FUNCTION_BLOCK FB_LD_IEDLD1 EXTENDS FB_AcsiCommonLogicalDeviceClass
VAR_INPUT
	LLN0: FB_LN_IED_LD1_LLN0 := (sClass:='LLN0', bLinkResult:=THIS^.AddLogicalNodeToContainer(ipLogicalNode:=LLN0));
	LPHD1: FB_LN_IED_LD1_LPHD1 := (sClass:='LPHD', bLinkResult:=THIS^.AddLogicalNodeToContainer(ipLogicalNode:=LPHD1));
	MMXU1: FB_LN_IED_LD1_MMXU1 := (sClass:='MMXU', bLinkResult:=THIS^.AddLogicalNodeToContainer(ipLogicalNode:=MMXU1));
	XCBR1: FB_LN_IED_LD1_XCBR1 := (sClass:='XCBR', bLinkResult:=THIS^.AddLogicalNodeToContainer(ipLogicalNode:=XCBR1));
	CSWI1: FB_LN_IED_LD1_CSWI1 := (sClass:='CSWI', bLinkResult:=THIS^.AddLogicalNodeToContainer(ipLogicalNode:=CSWI1));
	LEDGGIO1: FB_LN_IED_LD1_LEDGGIO1 := (sClass:='GGIO', bLinkResult:=THIS^.AddLogicalNodeToContainer(ipLogicalNode:=LEDGGIO1));
	LEDGGIO2: FB_LN_IED_LD1_LEDGGIO2 := (sClass:='GGIO', bLinkResult:=THIS^.AddLogicalNodeToContainer(ipLogicalNode:=LEDGGIO2));
	LEDGGIO3: FB_LN_IED_LD1_LEDGGIO3 := (sClass:='GGIO', bLinkResult:=THIS^.AddLogicalNodeToContainer(ipLogicalNode:=LEDGGIO3));
	LEDGGIO4: FB_LN_IED_LD1_LEDGGIO4 := (sClass:='GGIO', bLinkResult:=THIS^.AddLogicalNodeToContainer(ipLogicalNode:=LEDGGIO4));
	LEDGGIO5: FB_LN_IED_LD1_LEDGGIO5 := (sClass:='GGIO', bLinkResult:=THIS^.AddLogicalNodeToContainer(ipLogicalNode:=LEDGGIO5));
	LEDGGIO6: FB_LN_IED_LD1_LEDGGIO6 := (sClass:='GGIO', bLinkResult:=THIS^.AddLogicalNodeToContainer(ipLogicalNode:=LEDGGIO6));
	LEDGGIO7: FB_LN_IED_LD1_LEDGGIO7 := (sClass:='GGIO', bLinkResult:=THIS^.AddLogicalNodeToContainer(ipLogicalNode:=LEDGGIO7));
	LEDGGIO8: FB_LN_IED_LD1_LEDGGIO8 := (sClass:='GGIO', bLinkResult:=THIS^.AddLogicalNodeToContainer(ipLogicalNode:=LEDGGIO8));
	ATCC1: FB_LN_IED_LD1_ATCC1 := (sClass:='ATCC', bLinkResult:=THIS^.AddLogicalNodeToContainer(ipLogicalNode:=ATCC1));
END_VAR
VAR
END_VAR

END_FUNCTION_BLOCK
